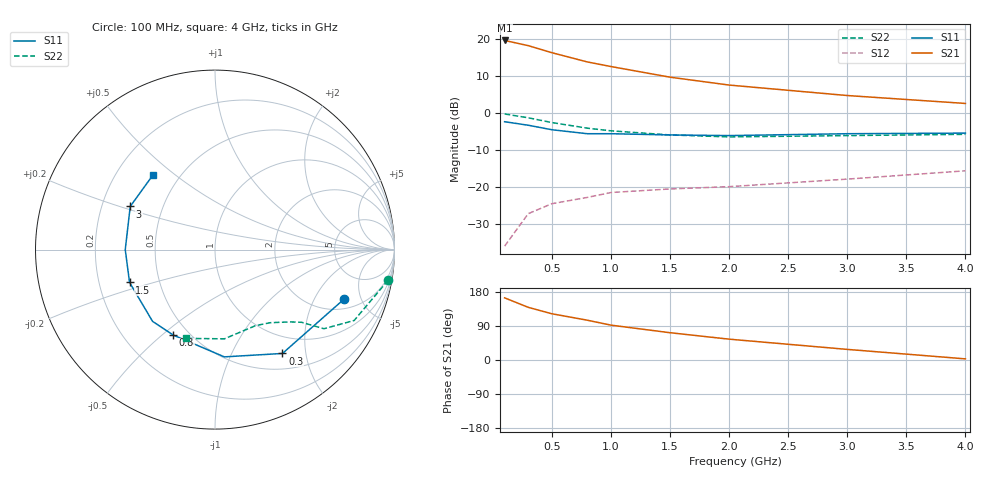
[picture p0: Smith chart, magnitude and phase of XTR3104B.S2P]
! HXTR-3104  (2N6839) Common Emitter
! Vce=10V  Ic=30mA
# ghz s ma r 50
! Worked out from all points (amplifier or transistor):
!   9 points, 100 MHz to 4 GHz, reference 50 ohm
!   highest |S21| = 19.7 dB at 100 MHz (marker M1)
!   |S21| within 3 dB of that: start of sweep to 467.6 MHz
!   unconditionally stable (mu >= 1): 1.777 GHz to 3.676 GHz
!   at 300 MHz: K = 0.24, MSG = 22.7 dB, |S12| = -27.1 dB
!   at 1 GHz: K = 0.68, MSG = 17.0 dB, |S12| = -21.4 dB
!   at 4 GHz: K = 0.97, MSG = 9.1 dB, |S12| = -15.5 dB
!   S11 on the Smith chart (normalised r, x): 100 MHz: 2.62, -3.56; 300 MHz: 0.72, -1.60; 800 MHz: 0.41, -0.55; 1.5 GHz: 0.33, -0.17; 3 GHz: 0.32, +0.22; 4 GHz: 0.36, +0.42
0.1  0.77 -21.0  9.66 164.0  0.016 71.0  0.98 -10.0
0.3  0.69 -57.0  8.22 139.0  0.044 58.0  0.87 -27.0
0.5  0.6 -85.0  6.6 122.0  0.06 48.0  0.75 -36.0
0.8  0.53 -116.0  4.95 105.0  0.073 40.0  0.63 -40.0
1  0.53 -131.0  4.29 92.0  0.085 34.0  0.58 -44.0
1.5  0.51 -159.0  3.08 72.0  0.095 32.0  0.51 -53.0
2  0.5 -180.0  2.41 55.0  0.102 31.0  0.48 -62.0
3  0.53 153.0  1.74 28.0  0.129 33.0  0.5 -84.0
4  0.54 130.0  1.36 3.0  0.167 29.0  0.52 -108.0
